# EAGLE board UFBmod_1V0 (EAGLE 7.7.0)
DL0WH Antenna BiTuner
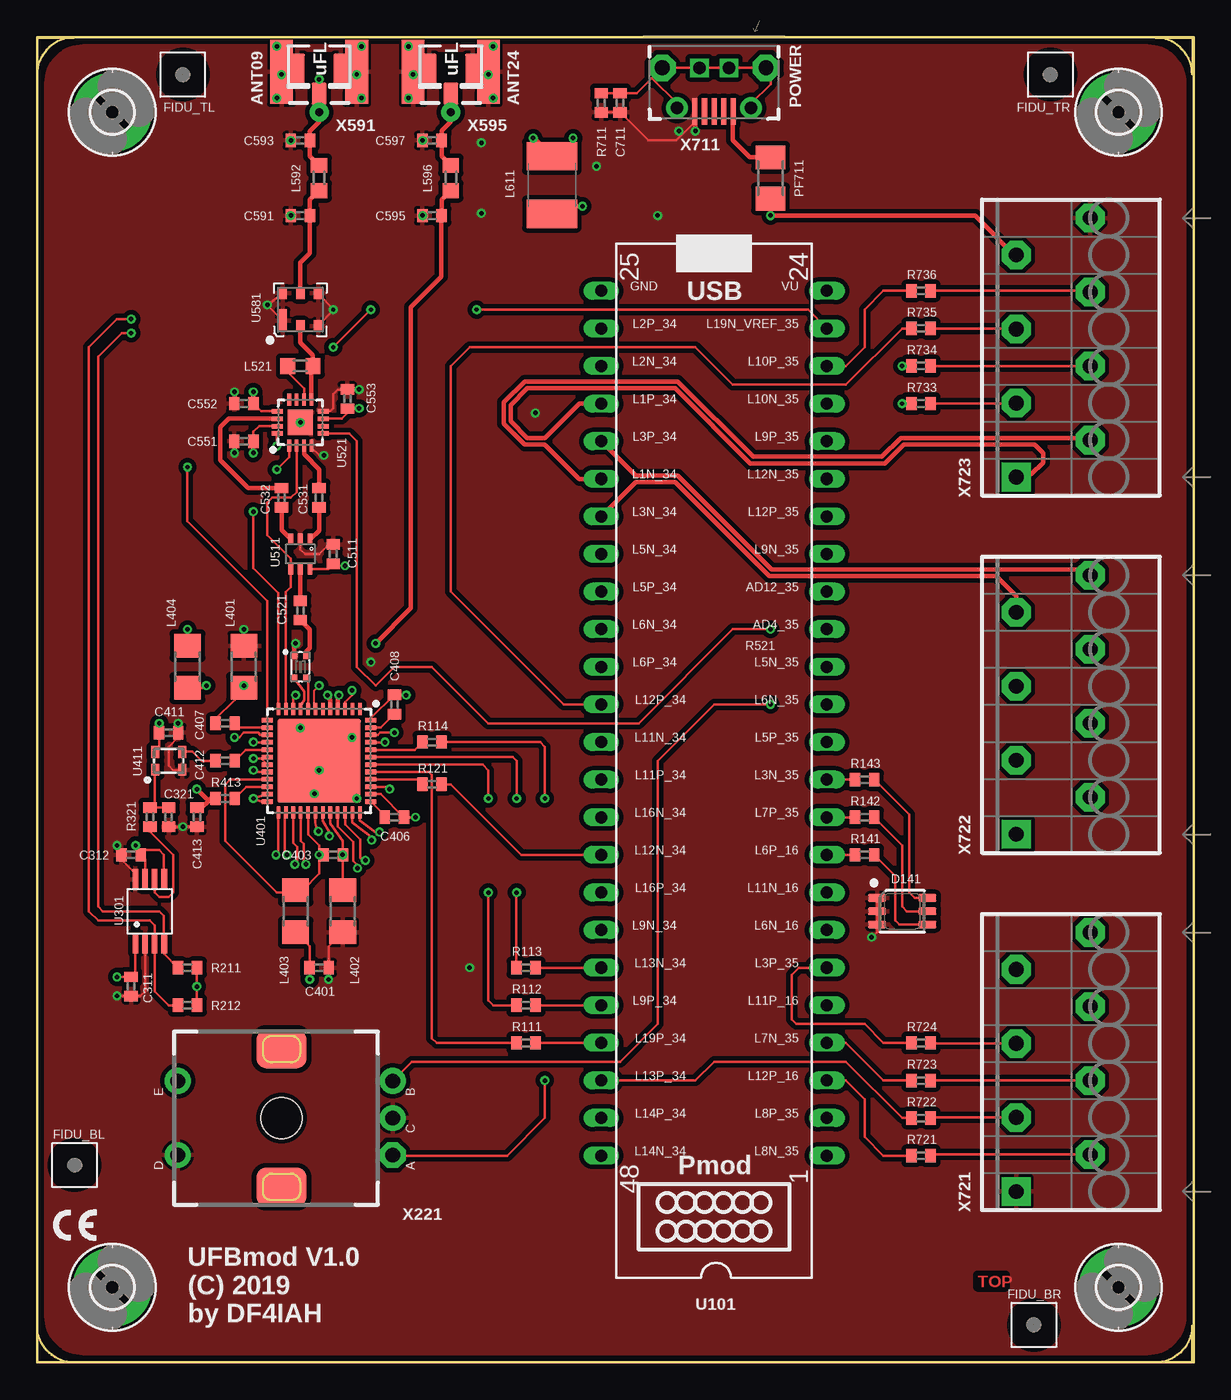
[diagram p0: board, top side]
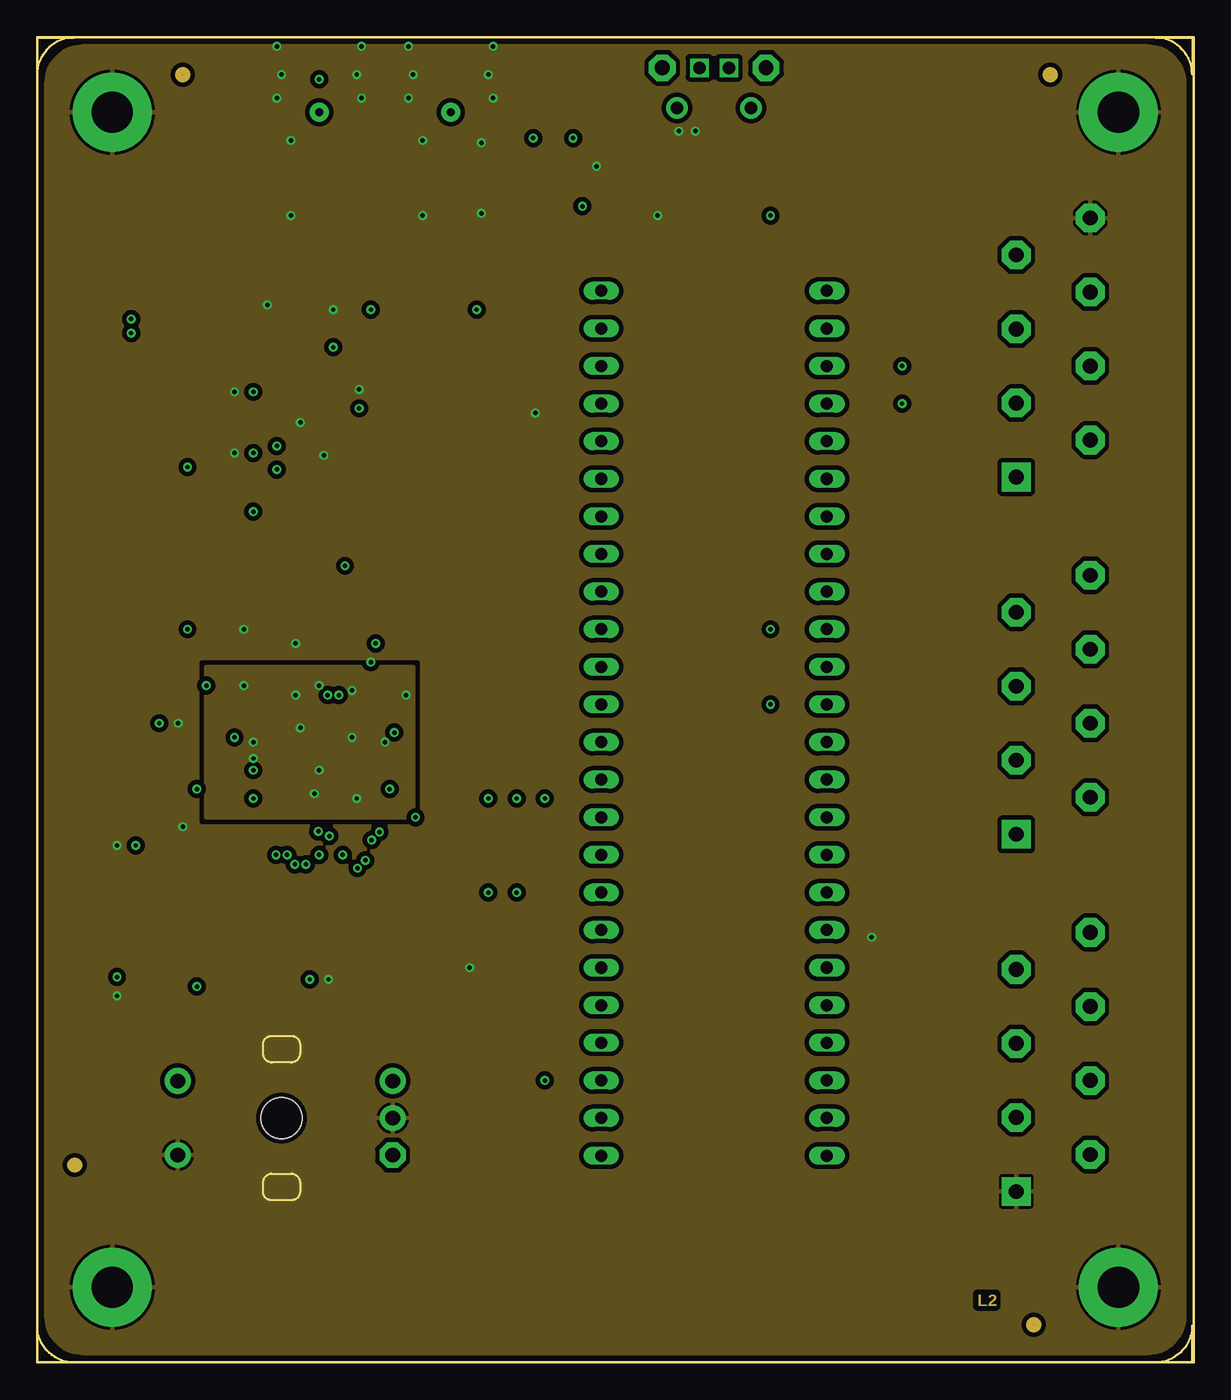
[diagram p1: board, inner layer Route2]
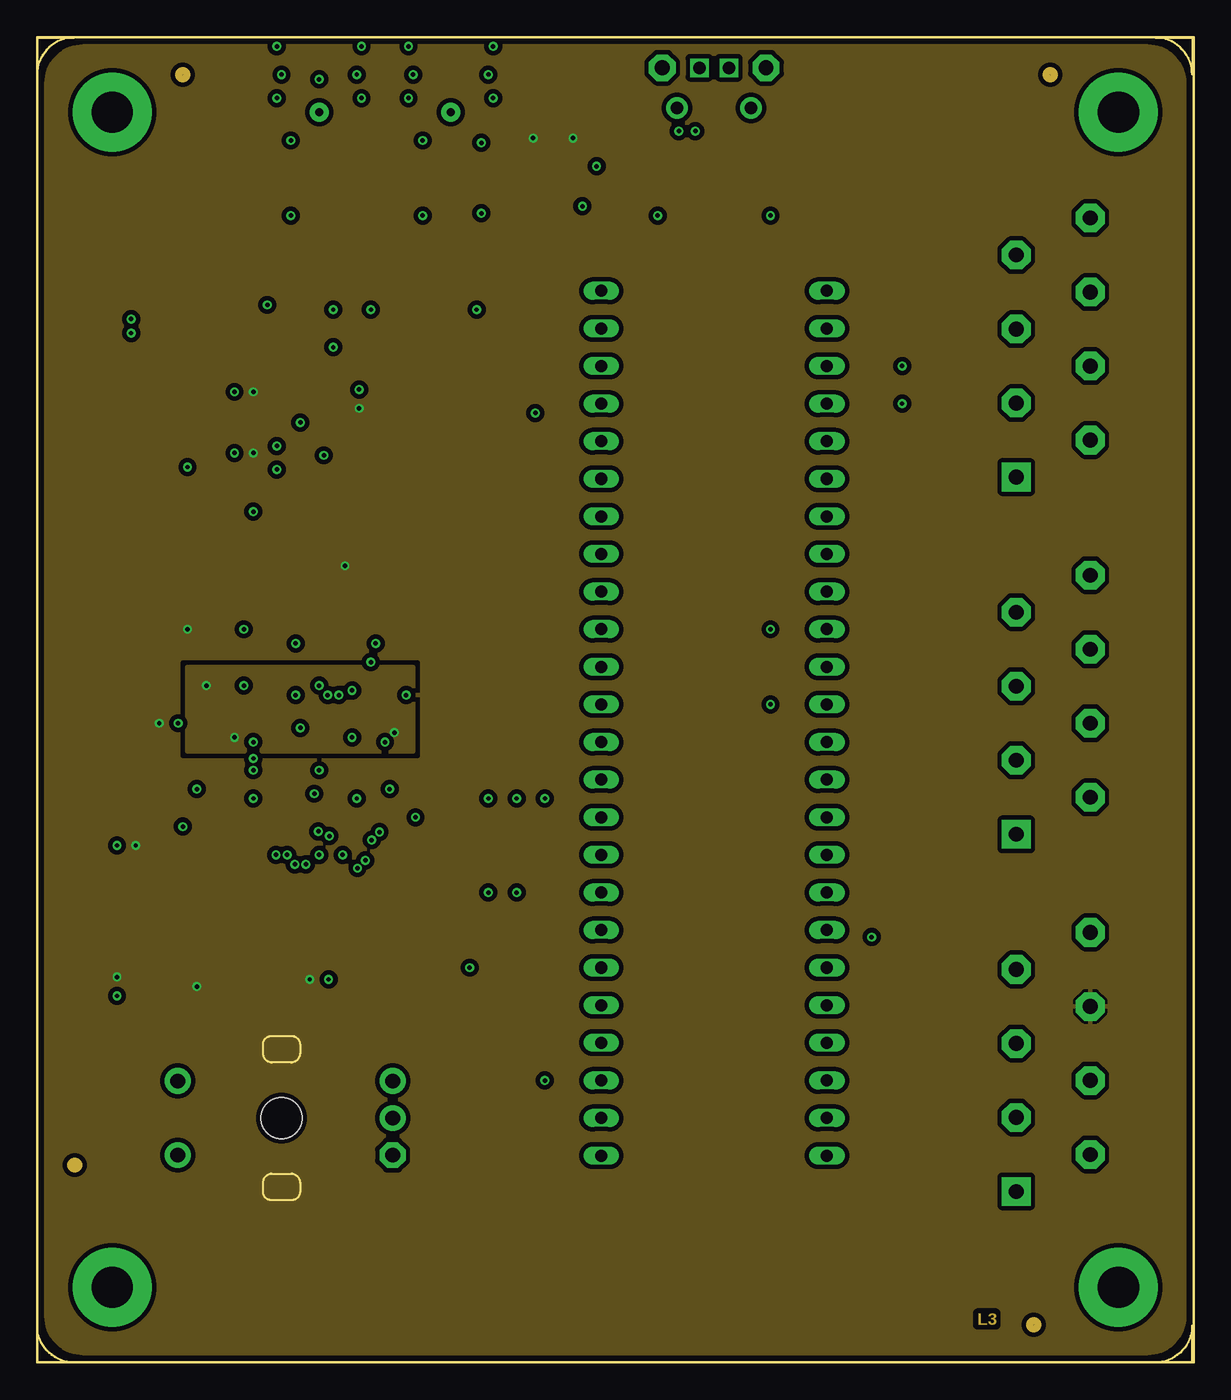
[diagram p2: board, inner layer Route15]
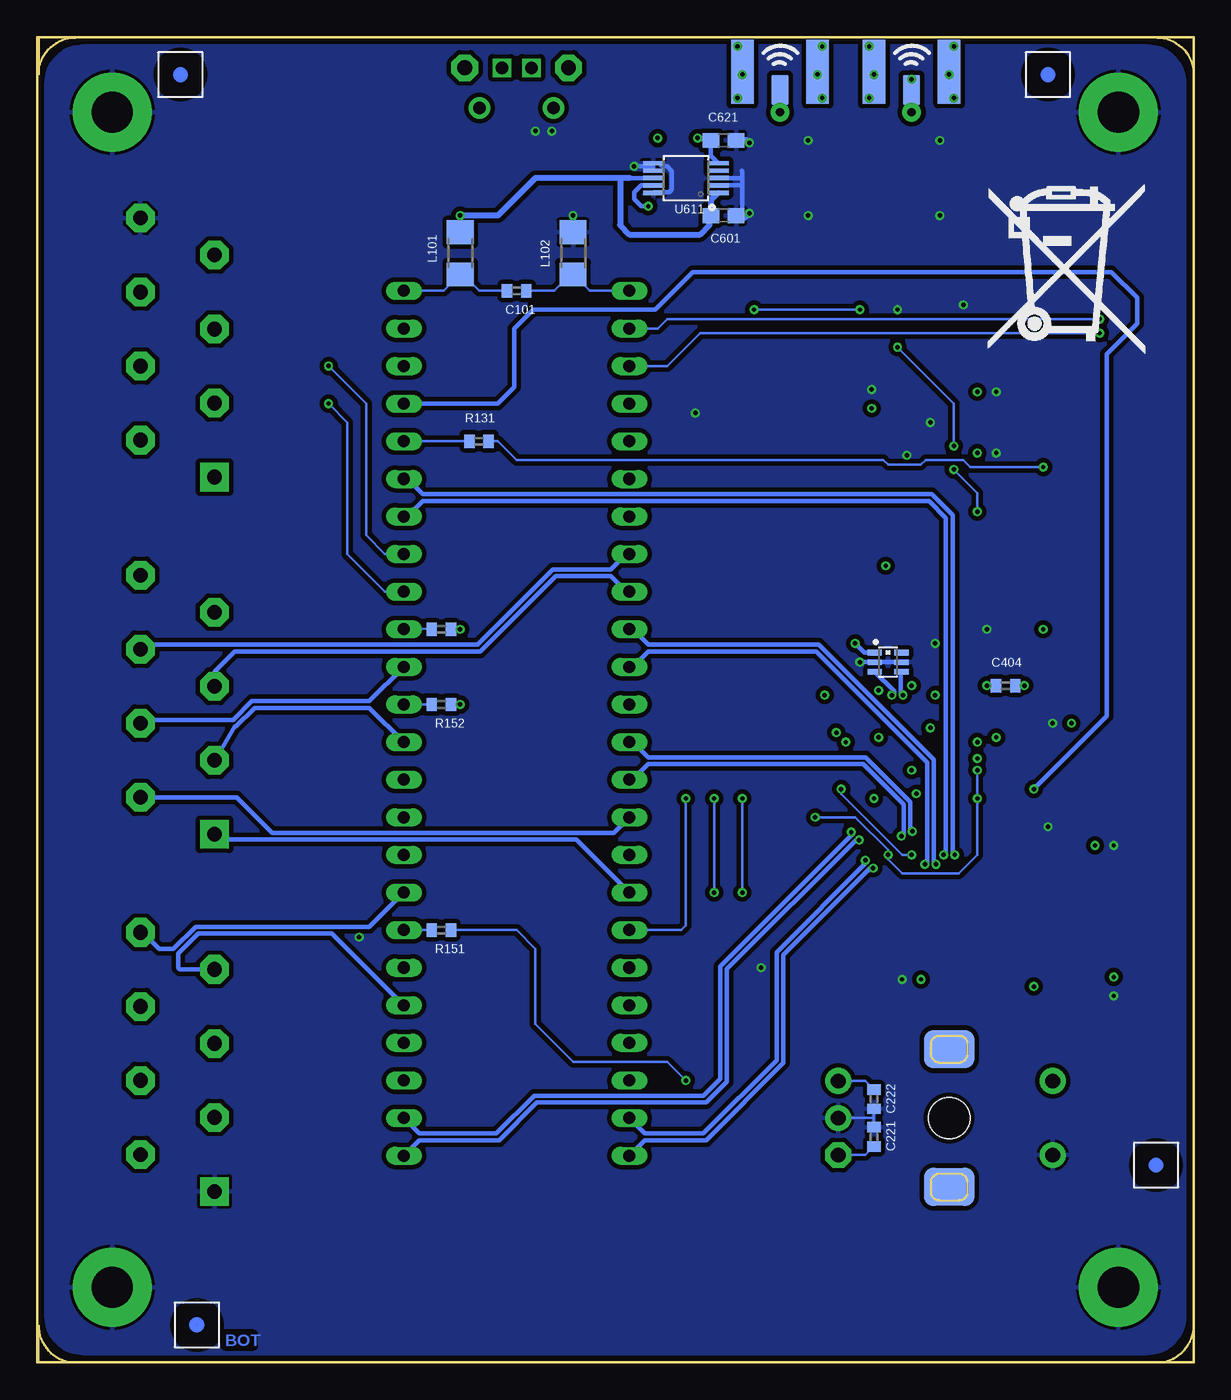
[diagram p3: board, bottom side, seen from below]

Size 78.11 x 89.53 mm. Coordinates in mm from the lower left corner, seen from the top.
Outline: 0,0 0,89.53 78.11,89.53 78.11,0 0,0
Copper layers (1+2*15+16): Top 0.035mm / dielectric 0.38mm / Route2 0.035mm / dielectric 0.71mm / Route15 0.035mm / dielectric 0.38mm / Bottom 0.035mm
Design rules "PCB-POOL Standard_ML4": minimum track width 0.15mm, minimum drill 0.3mm, track to track 0.15mm, track to pad 0.15mm, pad to pad 0.15mm, via to via 0.15mm, smd to smd 0.15mm, copper to edge 0.3mm, drill to drill 0.2mm, minimum pad ring 0.2mm, minimum via ring 0.15mm, stop-mask expansion 0.075mm, vias tented up to drill 0mil, thermal gap 0.2mm
Net classes: 0 default: drill 0.3 mm; 1 diff_100R: width 0.3 mm, clearance 0.15 mm; 2 pwr_ttl: width 0.75 mm, clearance 0.5 mm; 3 usb_pair: width 0.254 mm, clearance 0.152 mm; 4 pwrA5: width 0.4 mm; 5 single50R: width 0.838 mm, clearance 0.152 mm; 6 mil6_nofill: width 0.152 mm, clearance 0.254 mm
tRestrict: area 88.3,43.2 to 91.7,43.4; area 88.3,41.7 to 91.8,41.9; area 84.3,15.9 to 91.9,32.3
bRestrict: area 84.5,15.9 to 91.4,32.4; area 88.3,43.2 to 91.8,43.5; area 88.3,41.6 to 91.7,41.9; area 84.3,15.9 to 91.9,32.3
Milling: area 0,87 to 2.5,89.5; area 0,0 to 2.5,2.5; area 75.5,0 to 78,2.5; area 75.5,87 to 78,89.5

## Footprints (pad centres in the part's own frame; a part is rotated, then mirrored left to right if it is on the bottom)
C0402 = smd 0.7 x 0.9: 1 -0.65,0; 2 0.65,0
C0603 = smd 1.1 x 1: 1 -0.85,0; 2 0.85,0
ASMT-YTB7_0AA02_RGB = smd 1.2 x 0.5: 1 -1.7,0.9; 2 -1.7,0; 3 -1.7,-0.9; 4 1.7,-0.9; 5 1.7,0; 6 1.7,0.9
2,8-PAD = drill 2.8 pad 5.334: B2,8 0,0
R1206 = smd 1.6 x 1.803: 1 -1.422,0; 2 1.422,0
DXW21HN5011BL = smd 0.5 x 0.45: 1 -0.775,-0.4; 2 0.775,-0.4; 3 0.775,0.4; 4 -0.775,0.4
2450BL15B050 = smd 0.35 x 1: 1 -0.65,-0.9; 2 0,-0.9; 3 0.65,-0.9; 4 0.65,0.9; 5 0,0.9; 6 -0.65,0.9
L0603 = smd 1 x 1.1: 1 -0.85,0; 2 0.85,0
L1812 = smd 1.9 x 3.4: 1 -1.95,0; 2 1.95,0
M1206 = smd 1.6 x 2: 1 -1.4,0; 2 1.4,0
R0402 = smd 0.7 x 0.9: 1 -0.65,0; 2 0.65,0
DIGILENT_CMOD_A7__DIP48 = drill 0.813 long: 1 -29.21,-7.62; 2 -26.67,-7.62; 3 -24.13,-7.62; 4 -21.59,-7.62; 5 -19.05,-7.62; 6 -16.51,-7.62; 7 -13.97,-7.62; 8 -11.43,-7.62; 9 -8.89,-7.62; 10 -6.35,-7.62; 11 -3.81,-7.62; 12 -1.27,-7.62; 13 1.27,-7.62; 14 3.81,-7.62; 15 6.35,-7.62; 16 8.89,-7.62; 17 11.43,-7.62; 18 13.97,-7.62; 19 16.51,-7.62; 20 19.05,-7.62; 21 21.59,-7.62; 22 24.13,-7.62; 23 26.67,-7.62; 24 29.21,-7.62; 25 29.21,7.62; 26 26.67,7.62; 27 24.13,7.62; 28 21.59,7.62; 29 19.05,7.62; 30 16.51,7.62; 31 13.97,7.62; 32 11.43,7.62; 33 8.89,7.62; 34 6.35,7.62; 35 3.81,7.62; 36 1.27,7.62; 37 -1.27,7.62; 38 -3.81,7.62; 39 -6.35,7.62; 40 -8.89,7.62; 41 -11.43,7.62; 42 -13.97,7.62; 43 -16.51,7.62; 44 -19.05,7.62; 45 -21.59,7.62; 46 -24.13,7.62; 47 -26.67,7.62; 48 -29.21,7.62
µMAX8 = smd 1.35 x 0.4: 1 -2.15,0.975; 2 -2.15,0.325; 3 -2.15,-0.325; 4 -2.15,-0.975; 5 2.15,-0.975; 6 2.15,-0.325; 7 2.15,0.325; 8 2.15,0.975
QFN48_7X7-0P5-PAD = smd 0.8 x 0.3: 1 -3.5,2.75; 2 -3.5,2.25; 3 -3.5,1.75; 4 -3.5,1.25; 5 -3.5,0.75; 6 -3.5,0.25; 7 -3.5,-0.25; 8 -3.5,-0.75; 9 -3.5,-1.25; 10 -3.5,-1.75; 11 -3.5,-2.25; 12 -3.5,-2.75; 25 3.5,-2.75; 26 3.5,-2.25; 27 3.5,-1.75; 28 3.5,-1.25; 29 3.5,-0.75; 30 3.5,-0.25; 31 3.5,0.25; 32 3.5,0.75; 33 3.5,1.25; 34 3.5,1.75; 35 3.5,2.25; 36 3.5,2.75 | smd 0.3 x 0.8: 13 -2.75,-3.5; 14 -2.25,-3.5; 15 -1.75,-3.5; 16 -1.25,-3.5; 17 -0.75,-3.5; 18 -0.25,-3.5; 19 0.25,-3.5; 20 0.75,-3.5; 21 1.25,-3.5; 22 1.75,-3.5; 23 2.25,-3.5; 24 2.75,-3.5; 37 2.75,3.5; 38 2.25,3.5; 39 1.75,3.5; 40 1.25,3.5; 41 0.75,3.5; 42 0.25,3.5; 43 -0.25,3.5; 44 -0.75,3.5; 45 -1.25,3.5; 46 -1.75,3.5; 47 -2.25,3.5; 48 -2.75,3.5 | smd 5.65 x 5.65: 49 0,0
ASVTX-13 = smd 0.6 x 0.8: 1 -0.9,-0.6; 2 0.9,-0.6; 3 0.9,0.6; 4 -0.9,0.6
SC-70_6-LEAD_2X1MM25_0P65 = smd 0.4 x 0.8: 1 -0.65,-1; 2 0,-1; 3 0.65,-1; 4 0.65,1; 5 0,1; 6 -0.65,1
QFN16-3X3-0P5-PAD = smd 0.8 x 0.3: 1 -1.55,0.75; 2 -1.55,0.25; 3 -1.55,-0.25; 4 -1.55,-0.75; 9 1.55,-0.75; 10 1.55,-0.25; 11 1.55,0.25; 12 1.55,0.75 | smd 0.3 x 0.8: 5 -0.75,-1.55; 6 -0.25,-1.55; 7 0.25,-1.55; 8 0.75,-1.55; 13 0.75,1.55; 14 0.25,1.55; 15 -0.25,1.55; 16 -0.75,1.55 | smd 1.7 x 1.7: 17 0,0
B3440_3MM-X-3MM = smd 0.65 x 1.55: 1 -1.2,-0.75 | smd 0.65 x 0.8: 2 0,-1.125; 3 1.2,-1.125; 4 1.2,1.125; 5 0,1.125; 6 -1.2,1.125
S-PDSO-G10 = smd 0.3 x 1.45: 1 -1,-2.2; 2 -0.5,-2.2; 3 0,-2.2; 4 0.5,-2.2; 5 1,-2.2; 6 1,2.2; 7 0.5,2.2; 8 0,2.2; 9 -0.5,2.2; 10 -1,2.2
TTE_EN11-HSM = drill 1 pad 1.75 octagon: A -2.5,-7.5 | drill 1 pad 1.75: B 2.5,-7.5; C 0,-7.5; D -2.5,7; E 2.5,7 | smd 2.6 x 3.4: GND11 -4.65,0; GND12 4.65,0 | smd 2.6 x 3.4 bottom: GND21 -4.65,0; GND22 4.65,0 | hole 2.8: 0,0
SMA_UFL_PAD_TINY = smd 1.524 x 1.016: ANT1 -3.843,0 | drill 0.559 pad 1.27: ANT2 -5.08,0 | smd 2.032 x 1.143 bottom: ANT3 -3.589,0 | smd 2.2 x 1.016: GND1 -2.223,1.47; GND2 -2.223,-1.47 | smd 4.318 x 1.524: GND3 -2.349,-2.54; GND4 -2.349,2.54 | smd 4.318 x 1.524 bottom: GND5 -2.349,2.54; GND6 -2.349,-2.54
USB-B-MICRO-SMD_MOLEX-105017-0001 = smd 0.35 x 1.8: D+ 0,4.4; D- -0.65,4.4; GND 1.3,4.4; ID 0.65,4.4; VBUS -1.3,4.4 | drill 0.85 pad 1.45: JSHIELD -2.5,4.15; JSHIELD@2 2.5,4.15 | drill 1 pad 1.8 octagon: JSHIELD@3 -3.5,1.45; JSHIELD@6 3.5,1.45 | drill 0.85 square: JSHIELD@4 -1,1.45; JSHIELD@5 1,1.45
PHOENIX_1990067_1X8X2MM50_PTSA-0-5 = drill 1 pad 1.93 square: 1 -7.5,5 | drill 1 pad 1.93 octagon: 2 -5,0; 3 -2.5,5; 4 0,0; 5 2.5,5; 6 5,0; 7 7.5,5; 8 10,0

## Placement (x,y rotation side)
C101  100nF  [C0402]  45.72,72.39 180 bottom
C221  1nF  [C0402]  21.59,15.24 90 bottom
C222  1nF  [C0402]  21.59,17.78 270 bottom
C311  100nF  [C0402]  6.35,25.4 270 top
C312  100nF  [C0402]  6.35,34.29 180 top
C321  1uF  [C0402]  8.89,36.83 270 top
C401  1uF  [C0402]  19.05,26.67 0 top
C403  1nF  [C0402]  20,34.29 0 top
C404  1nF  [C0402]  12.7,45.72 180 bottom
C406  100nF  [C0402]  24.13,36.83 180 top
C407  100nF  [C0402]  12.7,43.18 0 top
C408  100nF  [C0402]  24.13,44.45 270 top
C411  10nF  [C0402]  8.89,42.55 0 top
C412  10nF  [C0402]  12.7,40.64 0 top
C413  56pF  [C0402]  10.79,36.83 270 top
C511  100nF  [C0402]  20,54.61 90 top
C521  1nF  [C0402]  17.78,50.8 270 top
C531  1nF  [C0402]  19.05,58.42 270 top
C532  1nF  [C0402]  16.51,58.42 270 top
C551  100nF  [C0402]  13.97,62.23 180 top
C552  100nF  [C0402]  13.97,64.77 180 top
C553  100nF  [C0402]  20.95,65.09 90 top
C591  0pF  [C0402]  17.78,77.47 180 top
C593  0pF  [C0402]  17.78,82.55 180 top
C595  0pF  [C0402]  26.67,77.47 180 top
C597  0pF  [C0402]  26.67,82.55 180 top
C601  10uF  [C0603]  31.75,77.47 0 bottom
C621  22uF  [C0603]  31.75,82.55 0 bottom
C711  1nF  [C0402]  39.37,85.09 90 top
D141  ASMT-YTB7-0AA02_RGB  [ASMT-YTB7_0AA02_RGB]  58.42,30.48 0 top
FIDU_BL  [FIDUCIAL_MARK_1MM]  2.54,13.34 0 top
FIDU_BR  [FIDUCIAL_MARK_1MM]  67.31,2.54 0 top
FIDU_TL  [FIDUCIAL_MARK_1MM]  9.84,87 0 top
FIDU_TR  [FIDUCIAL_MARK_1MM]  68.42,87 0 top
H2311  MOUNT-PAD-ROUND2.8  [2,8-PAD]  5.08,5.08 0 top
H2321  MOUNT-PAD-ROUND2.8  [2,8-PAD]  73.03,5.08 0 top
H2331  MOUNT-PAD-ROUND2.8  [2,8-PAD]  5.08,84.45 0 top
H2341  MOUNT-PAD-ROUND2.8  [2,8-PAD]  73.03,84.45 0 top
L101  300R  [R1206]  49.53,74.93 270 bottom
L102  300R  [R1206]  41.91,74.93 270 bottom
L401  300R  [R1206]  13.97,46.99 270 top
L402  300R  [R1206]  20.64,30.48 90 top
L403  300R  [R1206]  17.46,30.48 90 top
L404  300R  [R1206]  10.16,46.99 270 top
L421  MURATA DXW21HN5011BL  [DXW21HN5011BL]  17.78,46.99 270 top
L422  Johanson 2450BL15B050E  [2450BL15B050]  20.64,47.31 270 bottom
L521  ? nH  [L0603]  17.78,67.31 0 top
L592  0nH  [L0603]  19.05,80.01 90 top
L596  0nH  [L0603]  27.94,80.01 90 top
L611  10uH  [L1812]  34.77,79.53 270 top
PF711  1.1A/2.2A  [M1206]  49.53,80.01 90 top
R111  47R  [R0402]  33.02,21.59 180 top
R112  47R  [R0402]  33.02,24.13 180 top
R113  47R  [R0402]  33.02,26.67 180 top
R114  47R  [R0402]  26.67,41.91 180 top
R121  47R  [R0402]  26.67,39.05 180 top
R131  47R  [R0402]  48.26,62.23 180 bottom
R141  180R  [R0402]  55.88,34.29 180 top
R142  130R  [R0402]  55.88,36.83 180 top
R143  130R  [R0402]  55.88,39.37 180 top
R151  1kR  [R0402]  50.8,29.21 180 bottom
R152  1kR  [R0402]  50.8,44.45 180 bottom
R211  3.9kR  [R0402]  10.16,26.67 0 top
R212  3.9kR  [R0402]  10.16,24.13 0 top
R321  100kR  [R0402]  7.62,36.83 90 top
R413  100R  [R0402]  12.7,38.1 0 top
R521  1kR  [R0402]  50.8,49.53 180 bottom
R711  330kR  [R0402]  38.1,85.09 90 top
R721  100R  [R0402]  59.69,13.97 0 top
R722  100R  [R0402]  59.69,16.51 0 top
R723  100R  [R0402]  59.69,19.05 0 top
R724  100R  [R0402]  59.69,21.59 0 top
R733  100R  [R0402]  59.69,64.77 0 top
R734  100R  [R0402]  59.69,67.31 0 top
R735  100R  [R0402]  59.69,69.85 0 top
R736  100R  [R0402]  59.69,72.39 0 top
U101  DIGILENT_CMOD_A7  [DIGILENT_CMOD_A7__DIP48]  45.72,43.18 90 top
U301  MAX5217  [µMAX8]  7.62,30.48 90 top
U401  AT86RF215-ZU  [QFN48_7X7-0P5-PAD]  19.05,40.64 270 top
U411  ASVTX-13-D-26.000MHZ-I05-T  [ASVTX-13]  8.89,40.64 0 top
U511  PE4259  [SC-70_6-LEAD_2X1MM25_0P65]  17.78,54.61 180 top
U521  RFX1010  [QFN16-3X3-0P5-PAD]  17.78,63.5 90 top
U581  B39871B3440U410  [B3440_3MM-X-3MM]  17.78,71.12 0 top
U611  TPS62056DGSR  [S-PDSO-G10]  34.29,80.01 90 bottom
X221  TTE_EN11-HSM  [TTE_EN11-HSM]  16.51,16.51 90 top
X591  ANTENNATINY  [SMA_UFL_PAD_TINY]  19.05,89.53 90 top
X595  ANTENNATINY  [SMA_UFL_PAD_TINY]  27.94,89.53 90 top
X711  MOLEX 105017-0001  [USB-B-MICRO-SMD_MOLEX-105017-0001]  45.72,88.9 180 top
X721  PHOENIX_1990067_1X8X2MM50_PTSA-0-5  [PHOENIX_1990067_1X8X2MM50_PTSA-0-5]  71.12,19.05 90 top
X722  PHOENIX_1990067_1X8X2MM50_PTSA-0-5  [PHOENIX_1990067_1X8X2MM50_PTSA-0-5]  71.12,43.18 90 top
X723  PHOENIX_1990067_1X8X2MM50_PTSA-0-5  [PHOENIX_1990067_1X8X2MM50_PTSA-0-5]  71.12,67.31 90 top

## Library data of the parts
C101 C221 C222 C311 C312 C321 C401 C403 C404 C406-C408 C411-C413 C511 C521 C531 C532 C551-C553 C591 C593 C595 C597 C601 C621 C711 L101 L102 L401-L404 L521 L592 L596 L611 R111-R114 R121 R131 R141-R143 R151 R152 R211 R212 R321 R413 R521 R711 R721-R724 R733-R736 = df4iah_rcl
D141 = df4iah_led
FIDU_BL FIDU_BR FIDU_TL FIDU_TR = df4iah_fiducial
H2311 H2321 H2331 H2341 = df4iah_holes
L421 L422 = df4iah_balun
PF711 = rcl
U101 = df4iah_fpga
U301 = df4iah_dac
U401 U511 U521 U581 = df4iah_rf
U411 = df4iah_osc
U611 = df4iah_powersupply
X221 = df4iah_switch
X591 X595 = _c2h
X711 X721-X723 = df4iah_connector

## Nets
26MHZ_DAC_OUT: R321.1 U301.6
+3V3: C311.1 C312.1 C401.1 C411.1 C511.1 C551.1 C552.1 C553.1 C621.1 L403.1 L404.1 L611.1 R211.2 R212.2 U301.1 U301.5 U301.7 U411.4 U511.6 U521.7 U521.13 U521.15 U611.5 X721.6
+5V: C601.1 L101.1 PF711.1 U611.1 U611.8 X723.7
ANT09: C593.1 L592.2 X591.ANT1 X591.ANT2 X591.ANT3
ANT09_MATCH: C591.1 L592.1 U581.5
ANT24: C597.1 L596.2 X595.ANT1 X595.ANT2 X595.ANT3
FE09_ANT: L521.2 U521.9 U581.2
FE09_DET: R521.1 U521.5
FE09_IND: L521.1 U521.10
FE09_MODE: U101.23 U521.16
FE09_RX: C532.1 U521.14
FE09_TX: C531.1 U521.3
FPGA_1_34_N: U101.30 X723.2
FPGA_1_34_P: U101.28 X723.1
FPGA_3_34_N [diff_100R]: U101.29 X722.8
FPGA_3_34_P [diff_100R]: U101.31 X722.7
FPGA_3P35 [diff_100R]: R724.1 U101.6
FPGA_3P35_R [diff_100R]: R724.2 X721.5
FPGA_5_34_N [diff_100R]: U101.32 X722.6
FPGA_5_34_P [diff_100R]: U101.33 X722.5
FPGA_5_35_N [diff_100R]: U101.14 X722.4
FPGA_5_35_P [diff_100R]: U101.12 X722.3
FPGA_7N35 [diff_100R]: R723.1 U101.4
FPGA_7N35_R [diff_100R]: R723.2 X721.4
FPGA_9N35: R734.1 U101.17
FPGA_9N35_R: R734.2 X723.4
FPGA_10P35: R736.1 U101.22
FPGA_10P35_R: R736.2 X723.6
FPGA_11_16_N [diff_100R]: U101.8 X721.8
FPGA_11_16_P [diff_100R]: U101.5 X721.7
FPGA_12P16 [diff_100R]: R721.1 U101.3
FPGA_12P16_R [diff_100R]: R721.2 X721.2
FPGA_12P34: R735.1 U101.36
FPGA_12P34_R: R735.2 X723.5
FPGA_13P_34 [diff_100R]: R722.1 U101.46
FPGA_13P_34_R [diff_100R]: R722.2 X721.3
FPGA_16_34_N [diff_100R]: U101.39 X722.2
FPGA_16_34_P [diff_100R]: U101.41 X722.1
FPGA_AD12: R733.1 U101.16
FPGA_AD12_R: R733.2 X723.3
FPGA_FE09_DET: R521.2 U101.15
FPGA_I2C_SCL: R212.1 U101.26 U301.3
FPGA_I2C_SDA: R211.1 U101.27 U301.4
FPGA_MISO: R114.1 U101.42
FPGA_MOSI: R113.1 U101.43
FPGA_SCLK: R111.1 U101.45
FPGA_SELN: R112.1 U101.44
FPGA_TRX_CLKO: C413.1 R413.1 U101.21
FPGA_TRX_IRQ: R121.1 U101.40
FPGA_TRX_RSTN: R131.2 U101.20
GND: C221.2 C222.2 C311.2 C312.2 C321.2 C401.2 C411.2 C413.2 C511.2 C551.2 C552.2 C553.2 C591.2 C593.2 C595.2 C597.2 C601.2 C621.2 C711.1 D141.1 D141.2 D141.3 H2311.B2,8 H2321.B2,8 H2331.B2,8 H2341.B2,8 L102.1 L401.1 L402.1 L421.1 L422.2 L422.5 R711.1 U301.2 U301.8 U411.2 U511.2 U521.4 U521.8 U521.17 U581.1 U581.3 U581.4 U581.6 U611.3 U611.6 U611.7 U611.10 X221.C X221.D X591.GND1 X591.GND2 X591.GND3 X591.GND4 X595.GND1 X595.GND2 X595.GND3 X595.GND4 X711.GND X721.1 X723.8
LED_B: D141.6 R143.1
LED_B_R: R143.2 U101.11
LED_G: D141.5 R142.1
LED_G_R: R142.2 U101.10
LED_R: D141.4 R141.1
LED_R_R: R141.2 U101.9
PE09_RF1: C531.2 U511.1
PE09_RF2: C532.2 U511.3
PE09_RFC: C521.1 U511.5
PMIC3V3_SW: L611.2 U611.9
ROT_I: R151.2 U101.7
ROT_I_R: C221.1 R151.1 X221.A
ROT_Q: R152.2 U101.13
ROT_Q_R: C222.1 R152.1 X221.B
TRX_AVDD0: C407.2 U401.14
TRX_AVDD1: C408.2 U401.47
TRX_AVSS: C404.2 C407.1 C408.1 L401.2 U401.3 U401.6 U401.7 U401.10 U401.16 U401.18 U401.19 U401.45 U401.48 U401.49
TRX_CLKO: R413.2 U401.22
TRX_DEVDD: C403.1 L403.2 U401.21 U401.29 U401.39
TRX_DVDD: C406.2 U401.37
TRX_DVSS: C403.2 C406.1 L402.2 U401.20 U401.23 U401.24 U401.32 U401.38
TRX_EVDD: C404.1 L404.2 U401.15 U401.46
TRX_FEA09: U401.11 U511.4 U521.2
TRX_FEA24: U401.1
TRX_FEB09: U401.12 U521.1
TRX_FEB24: U401.2
TRX_IRQ: R121.2 U401.40
TRX_MISO: R114.2 U401.44
TRX_MOSI: R113.2 U401.43
TRX_RF09: C521.2 L421.4
TRX_RF09_N [diff_100R]: L421.2 U401.9
TRX_RF09_P [diff_100R]: L421.3 U401.8
TRX_RF24: C595.1 L422.1 L596.1
TRX_RF24_N: L422.4 U401.5
TRX_RF24_P: L422.3 U401.4
TRX_RSTN: R131.1 U401.13
TRX_RXCLK_N [diff_100R]: U101.48 U401.33
TRX_RXCLK_P [diff_100R]: U101.47 U401.34
TRX_RXD09_N [diff_100R]: U101.37 U401.30
TRX_RXD09_P [diff_100R]: U101.38 U401.31
TRX_RXD24_N [diff_100R]: U101.1 U401.35
TRX_RXD24_P [diff_100R]: U101.2 U401.36
TRX_SCLK: R111.2 U401.41
TRX_SELN: R112.2 U401.42
TRX_TCXO: C412.2 U401.17
TRX_TXCLK_N [diff_100R]: U101.19 U401.25
TRX_TXCLK_P [diff_100R]: U101.18 U401.26
TRX_TXD_N [diff_100R]: U101.34 U401.27
TRX_TXD_P [diff_100R]: U101.35 U401.28
USB_SHIELD: C711.2 R711.2 X711.JSHIELD X711.JSHIELD@2 X711.JSHIELD@3 X711.JSHIELD@4 X711.JSHIELD@5 X711.JSHIELD@6
USB_VBUS: PF711.2 X711.VBUS
VCCA: C101.2 L101.2 U101.24
VCTCXO_OUT: C412.1 U411.3
VCTCXO_VC: C321.1 R321.2 U411.1
VSSA: C101.1 L102.2 U101.25

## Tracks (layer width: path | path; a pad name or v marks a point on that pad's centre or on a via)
26MHZ_DAC_OUT
  Top 0.152: U301.6 7.94,32.64 7.94,31.75 8.26,31.43 8.89,31.43 9.21,31.75 9.21,34.29 7.62,35.88 R321.1
+3V3  (via drill 0.3)
  Top 0.15: 34.61,81.76 arc45 34.69,81.56 L611.1 | C511.1 20.15,53.82 v20.8,53.82
  Top 0.152: L403.1 18.4,28.12 C401.1 18.4,26.05 v18.41,25.88 | R211.2 10.79,26.66 v10.79,25.4 10.79,24.14 R212.2 | v5.4,26.04 6.33,26.04 C311.1 6.64,26.34 U301.1 | U301.7 7.3,32.64 7.3,33.97 7,34.27 C312.1 7,34.62 | U301.5 8.57,32.65 8.57,34.29 8.26,34.61 7.3,34.61 7,34.62 | 7,34.62 6.7,34.92 v6.67,34.92 | v8.26,43.18 8.26,42.56 C411.1 8.24,41.49 U411.4 | L404.1 v10.16,49.53 | U511.6 19.65,53.61 C511.1 | U521.13 15.14,64.25 C552.1 | U521.15 14.99,63.25 14.61,62.87 14.61,62.24 C551.1 | U521.7 20.57,63.75 20.95,64.14 C553.1 20.97,64.45 v21.75,64.45
  Top 0.3: v14.61,65.56 14.61,64.78 C552.1 | v14.61,61.44 14.61,62.22 C551.1 | 34.61,81.76 35.08,82.23 36.04,82.23 36.2,82.39 v36.2,82.71
  Top 0.406: 34.61,81.76 34.45,81.76 v33.5,82.71
  Bottom 0.15: 32.54,82.55 C621.1
  Bottom 0.3: U611.5 32.6,81.52 C621.1
  Bottom 0.406: v33.5,82.71 32.7,82.71 32.54,82.55
  pour Route15 (isolate 0.305, rank 2): 74.97,0.64 3.13,0.64 arc-90 0.64,3.13 0.64,86.4 arc-90 3.13,88.9 74.97,88.9 arc-90 77.47,86.4 77.47,3.13 arc-90
+5V  (via drill 0.3)
  Top 0.3: PF711.1 v49.53,77.47 63.34,77.47 66,74.81 X723.7
  Bottom 0.15: 32.7,77.47 C601.1
  Bottom 0.3: L101.1 v49.53,77.47 | U611.8 38.1,80.01
  Bottom 0.406: 38.1,80.01 38.73,80.01 | 38.73,80.01 44.45,80.01 46.99,77.47 v49.53,77.47 | U611.1 32.6,78.5 C601.1 | 38.73,80.01 38.73,76.83 38.1,76.2 33.34,76.2 32.7,76.83 32.7,77.47
ANT09  (via drill 0.3)
  Top 0.3: C593.1 18.43,81.48 L592.2 | 18.41,82.56 18.41,83.19 19.05,83.82 X591.ANT2 X591.ANT1 v19.05,86.68
  Top 0.406: 18.41,82.56 C593.1
  Bottom 0.3: X591.ANT3 v19.05,86.68
ANT09_MATCH
  Top 0.3: C591.1 18.43,78.54 L592.1 | U581.5 17.78,74.3 18.41,74.93 18.41,77.45
  Top 0.406: 18.41,77.45 C591.1
ANT24
  Top 0.3: L596.2 27.32,81.48 C597.1 27.32,83.2 27.94,83.82 X595.ANT2 X595.ANT1
  Bottom 0.3: X595.ANT3 X595.ANT2
FE09_ANT
  Top 0.3: U521.9 18.53,67.21 | L521.2 18.63,68.05 17.78,68.9 U581.2
  Top 0.406: 18.53,67.21 L521.2
FE09_DET  (via drill 0.3)
  Top 0.152: v49.53,49.53 46.99,49.53 40.64,43.18 30.48,43.18 26.67,46.99 24.13,46.99 22.86,45.72 21.59,46.99 21.59,62.23 21.07,62.75 U521.5
  Bottom 0.152: R521.1 v49.53,49.53
FE09_IND
  Top 0.152: U521.10 18.03,65.79 16.93,66.89 L521.1
FE09_MODE  (via drill 0.3)
  Top 0.152: U101.23 52.07,71.12 v29.69,71.12 | v22.54,71.12 v20,68.58 | U521.16 16.19,62.71 v16.19,61.91
  Bottom 0.152: v29.69,71.12 v22.54,71.12 | v16.19,61.91 16.19,64.77 v20,68.58
FE09_RX
  Top 0.3: C532.1 14.27,59.07 12.38,60.96 12.38,63.18 12.95,63.75 U521.14
FE09_TX
  Top 0.3: U521.3 18.03,61.34 19.05,60.33 C531.1
FPGA_1_34_N
  Top 0.3: U101.30 36.6,59.69 34.29,62.01 32.93,62.01 31.52,63.41 31.52,64.86 32.93,66.27 43.27,66.27 48.35,61.19 57.06,61.19 58.33,62.45 70.97,62.45 X723.2
FPGA_1_34_P
  Top 0.3: U101.28 36.6,64.77 34.29,62.45 33.11,62.45 31.98,63.59 31.98,64.68 33.11,65.81 43.09,65.81 48.17,60.73 57.24,60.73 58.51,62.01 67.38,62.01 67.94,61.44 67.94,60.8 67.15,60.01 66.32,60.01 X723.1
FPGA_3_34_N
  Top 0.3: U101.29 40.41,59.91 43.27,59.91 49.62,53.56 70.73,53.56 X722.8
FPGA_3_34_P
  Top 0.3: U101.31 40.41,59.47 43.09,59.47 49.44,53.12 64.77,53.12 66.12,51.77 X722.7
FPGA_3P35
  Top 0.152: U101.6 51.44,26.67 50.96,26.19 50.96,23.18 51.28,22.86 55.88,22.86 57.15,21.59 R724.1
FPGA_3P35_R
  Top 0.152: 60.38,21.55 X721.5
  Top 0.3: R724.2 60.38,21.55
FPGA_5_34_N
  Bottom 0.3: U101.32 38.33,54.61 39.37,53.56 43.27,53.56 48.35,48.48 70.81,48.48 X722.6
FPGA_5_34_P
  Bottom 0.3: U101.33 38.33,52.07 39.37,53.12 43.09,53.12 48.17,48.03 64.77,48.03 66.12,46.69 X722.5
FPGA_5_35_N
  Bottom 0.3: U101.14 55.66,44.67 63.59,44.67 64.86,43.41 70.89,43.41 arc-90 X722.4
FPGA_5_35_P
  Bottom 0.3: U101.12 55.66,44.23 63.41,44.23 64.68,42.95 64.77,42.95 66.04,40.76 arc90 X722.3
FPGA_7N35
  Top 0.152: U101.4 54.61,21.59 57.15,19.05 R723.1
FPGA_7N35_R
  Top 0.152: R723.2 X721.4
FPGA_9N35  (via drill 0.3)
  Top 0.152: v58.42,67.31 R734.1
  Bottom 0.152: U101.17 54.61,54.61 55.88,55.88 55.88,64.77 v58.42,67.31
FPGA_9N35_R
  Top 0.152: R734.2 X723.4
FPGA_10P35
  Top 0.152: U101.22 54.61,67.31 55.88,68.58 55.88,71.12 57.15,72.39 R736.1
FPGA_10P35_R
  Top 0.152: R736.2 71.04,72.39
  Top 0.3: 71.04,72.39 X723.6
FPGA_11_16_N
  Bottom 0.3: U101.8 55.66,29.43 67.4,29.43 68.9,27.94 69.85,27.94 70.96,29.05 X721.8
FPGA_11_16_P
  Bottom 0.3: U101.5 58.2,28.98 67.22,28.98 68.58,27.62 68.58,26.67 68.46,26.55 X721.7
FPGA_12P16
  Top 0.152: U101.3 54.61,19.05 55.88,17.78 55.88,15.24 57.15,13.97 R721.1
FPGA_12P16_R
  Top 0.152: 60.42,14.05 X721.2
  Top 0.3: R721.2 60.42,14.05
FPGA_12P34
  Top 0.152: U101.36 35.56,44.45 27.94,52.07 27.94,67.31 29.21,68.58 44.45,68.58 46.99,66.04 54.61,66.04 58.42,69.85 R735.1
FPGA_12P34_R
  Top 0.152: R735.2 66.08,69.85
  Top 0.3: 66.08,69.85 X723.5
FPGA_13P_34
  Top 0.152: U101.46 44.45,19.05 45.72,20.32 54.61,20.32 58.42,16.51 R722.1
FPGA_13P_34_R
  Top 0.152: 60.38,16.55 X721.3
  Top 0.3: R722.2 60.38,16.55
FPGA_16_34_N
  Bottom 0.3: U101.39 39.15,35.78 62.23,35.78 64.62,38.18 X722.2
FPGA_16_34_P
  Bottom 0.3: U101.41 41.69,35.34 65.78,35.34 X722.1
FPGA_AD12  (via drill 0.3)
  Top 0.152: v58.42,64.77 R733.1
  Bottom 0.152: U101.16 54.61,52.07 57.15,54.61 57.15,63.5 v58.42,64.77
FPGA_AD12_R
  Top 0.152: R733.2 66.08,64.77 X723.3
FPGA_FE09_DET
  Bottom 0.15: R521.2 U101.15
FPGA_I2C_SCL  (via drill 0.3)
  Top 0.152: R212.1 8.89,24.13 7.95,25.07 U301.3 7.94,28.34 7.94,29.53 7.62,29.84 4.13,29.84 3.49,30.48 3.49,68.58 5.4,70.48 v6.35,70.48
  Bottom 0.152: U101.26 36.2,69.85 35.56,70.48 v6.35,70.48
FPGA_I2C_SDA  (via drill 0.3)
  Top 0.152: R211.1 8.6,27.59 U301.4 8.57,28.35 8.57,30.16 8.26,30.48 4.45,30.48 4.13,30.8 4.13,67.94 5.71,69.53 v6.35,69.53
  Bottom 0.152: U101.27 35.56,67.31 33.34,69.53 v6.35,69.53
FPGA_MISO  (via drill 0.3)
  Top 0.152: R114.1 33.97,41.91 34.29,41.59 v34.29,38.1
  Bottom 0.152: U101.42 34.61,29.21 34.29,29.53 v34.29,38.1
FPGA_MOSI
  Top 0.152: U101.43 R113.1
FPGA_SCLK
  Top 0.152: U101.45 R111.1
FPGA_SELN
  Top 0.152: U101.44 R112.1
FPGA_TRX_CLKO  (via drill 0.3)
  Top 0.152: R413.1 11.75,38.1 | 11.13,37.48 C413.1
  Top 0.3: 11.75,38.1 11.59,37.94 | 11.59,37.94 11.13,37.48 | v10.79,38.73 11.59,37.94
  Bottom 0.3: v10.79,38.73 5.87,43.66 5.87,68.1 3.81,70.17 3.81,71.91 5.56,73.66 33.81,73.66 36.35,71.12 44.61,71.12 45.88,69.85 45.88,65.88 46.99,64.77 U101.21
FPGA_TRX_IRQ
  Top 0.152: R121.1 27.94,39.05 32.7,34.29 U101.40
FPGA_TRX_RSTN
  Bottom 0.152: R131.2 U101.20
GND  (via drill 0.3)
  Top 0.152: X711.GND 44.42,83.79 43.18,82.55 41.26,82.55 C711.1 R711.1 | L402.1 19.7,28.12 C401.2 19.7,26.05 v19.68,25.88 | v5.4,24.77 6.33,24.77 C311.2 6.37,24.77 6.99,24.77 7.29,25.07 U301.2 | U301.8 6.64,33.04 5.7,33.99 C312.2 5.4,34.59 v5.4,34.92 | C321.2 C413.2 10.78,36.2 v9.84,36.2 | v9.53,43.18 9.53,42.56 C411.2 9.54,42.24 8.89,41.59 8.89,40.32 9.21,40.01 9.76,40.01 U411.2 | L401.1 v13.97,49.53 | U511.2 17.78,54.93 18.1,54.61 19.05,54.61 19.7,55.26 | U581.4 19.05,72.17 v20,71.12 19.05,70.06 U581.3 | U581.6 16.51,72.17 v15.56,71.44 15.63,71.37 U581.1 | U521.8 19.8,64.25 20,64.45 20,65.41 20.32,65.72 20.94,65.72 C553.2 21.57,65.74 v21.75,65.72 | U521.4 18.53,61.8 19.05,61.28 v19.37,61.28 | v17.14,77.47 C591.2 | v17.14,82.55 C593.2 | D141.1 D141.2 D141.3 56.72,29.1 v56.36,28.73
  Top 0.3: L421.1 17.38,48.49 v17.46,48.58 | 19.7,55.26 C511.2 | v13.34,65.56 13.34,64.78 C552.2 | v13.34,61.44 13.34,62.22 C551.2 | v16.19,88.9 16.19,87.5 X591.GND4 17.45,87.19 X591.GND1 | v16.51,87 16.19,86.68 v16.19,85.41 | v21.91,88.9 21.91,87.5 X591.GND3 20.65,87.19 X591.GND2 | v21.91,85.41 21.59,85.72 v21.59,87 | 44.42,83.79 44.45,83.76 v44.45,83.19 | X595.GND4 25.4,88.58 v25.08,88.9 | v25.08,85.41 25.4,85.72 v25.4,87 X595.GND4 | v30.8,85.41 30.8,86.68 v30.48,87 X595.GND3 | v30.8,88.9 30.8,87.5 X595.GND3 | X595.GND1 25.53,87.31 X595.GND4 | X595.GND2 30.35,87.31 X595.GND3
  Bottom 0.15: 31.43,80.01 U611.3
  Bottom 0.152: 41.91,76.52 v41.91,77.47 | C221.2 21.59,16.51 | 21.59,16.51 C222.2 | X221.C 21.59,16.51
  Bottom 0.3: v22.54,47.31 L422.2 L422.5 | C601.2 30.48,77.89 30.48,79.53 | 30.48,79.53 30.48,80.01 | 30.48,80.01 30.48,80.49 30.5,80.51 | 30.48,80.01 31.43,80.01 | 30.48,79.53 31.43,79.53 | U611.6 36.7,80.8 v37.78,80.8 | U611.10 36.44,79.06 35.4,79.06 35.24,79.22 35.24,80.49 35.56,80.8 35.88,80.8 36.08,81.01 U611.6 | U611.7 U611.6
  Bottom 0.406: v30,82.39 30.16,82.55 30.96,82.55 | v30,77.63 30.32,77.31 30.8,77.31
  other vias: 17.78,63.5 26.04,82.55 26.04,77.47 29.21,26.67 33.66,64.14 43.34,83.19
  pour Top (isolate 0.305): 74.97,0.64 3.13,0.64 arc-90 0.64,3.13 0.64,86.4 arc-90 3.13,88.9 74.97,88.9 arc-90 77.47,86.4 77.47,3.13 arc-90
  pour Route2 (isolate 0.305, rank 2): 74.97,0.64 3.13,0.64 arc-90 0.64,3.13 0.64,86.4 arc-90 3.13,88.9 74.97,88.9 arc-90 77.47,86.4 77.47,3.13 arc-90
  pour Bottom (isolate 0.305): 74.97,0.64 3.13,0.64 arc-90 0.64,3.13 0.64,86.4 arc-90 3.13,88.9 74.97,88.9 arc-90 77.47,86.4 77.47,3.13 arc-90
LED_B
  Top 0.152: D141.6 59.27,31.38 58.9,31.75 58.9,37 R143.1
LED_B_R
  Top 0.152: U101.11 R143.2
LED_G
  Top 0.152: D141.5 58.74,30.48 58.42,30.8 58.42,34.94 R142.1
LED_G_R
  Top 0.152: U101.10 R142.2
LED_R
  Top 0.152: D141.4 58.21,29.58 57.94,29.84 57.94,32.88 R141.1
LED_R_R
  Top 0.152: U101.9 R141.2
PE09_RF1
  Top 0.3: U511.1 18.46,55.61 19.05,56.2 C531.2
PE09_RF2
  Top 0.3: C532.2 16.51,56.23 U511.3
PE09_RFC
  Top 0.3: U511.5 C521.1
PMIC3V3_SW  (via drill 0.3)
  Top 0.3: L611.2 35.29,78.11 v36.83,78.11
  Bottom 0.3: U611.9 36.51,79.53 37.31,79.53 37.78,79.06 37.78,78.58 37.31,78.11 v36.83,78.11
ROT_I
  Bottom 0.152: U101.7 R151.2
ROT_I_R  (via drill 0.3)
  Top 0.152: X221.A 24.05,13.97 31.75,13.97 34.29,16.51 v34.29,19.05
  Bottom 0.152: C221.1 22.17,14.01 X221.A | v34.29,19.05 35.56,20.32 41.91,20.32 44.45,22.86 44.45,27.94 45.72,29.21 R151.1
ROT_Q
  Bottom 0.152: U101.13 R152.2
ROT_Q_R  (via drill 0.3)
  Top 0.152: X221.B 25.32,20.32 39.37,20.32 41.91,22.86 41.91,40.64 45.72,44.45 v49.53,44.45
  Bottom 0.152: C222.1 22.17,19.01 X221.B | v49.53,44.45 R152.1
TRX_AVDD0
  Top 0.152: U401.14 13.64,42.89 C407.2
TRX_AVDD1
  Top 0.152: C408.2 23.22,42.89 U401.47
TRX_AVSS  (via drill 0.3)
  Top 0.15: U401.6 U401.7 18.73,44.21 18.73,45.4 v19.05,45.72
  Top 0.152: U401.48 22.55,43.52 C408.1 24.46,45.1 v24.92,45.09 | U401.3 20.8,44.61 21.27,45.09 v21.27,45.4 | v21.59,38.1 v18.73,38.42 19.05,38.42 v19.05,40.01 U401.49 19.05,41.59 v17.78,42.86 20.64,42.86 v21.27,42.23 | U401.10 17.3,44.92 v17.46,45.09 | v13.97,45.72 L401.2 13.34,44.93 13.34,44.77 12.05,43.48 C407.1 | U401.45 23.48,41.89 v23.5,41.91 | U401.16 14.62,41.89 v14.61,41.91 | U401.18 15.46,40.8 v14.61,40.8 15.14,40.8 U401.19
  Bottom 0.152: C404.2 13.35,45.7 v13.97,45.72
  pour Route2 (isolate 0.305): 11.43,46.99 25.4,46.99 25.4,36.83 11.43,36.83
TRX_CLKO
  Top 0.152: U401.22 14.14,38.89 R413.2
TRX_DEVDD  (via drill 0.3)
  Top 0.152: U401.29 18.3,35.67 19.05,34.92 v19.05,34.29 | v19.05,34.29 C403.1 | v19.05,34.29 19.05,33.02 17.93,31.9 L403.2 17.31,31.75 16.19,31.75 12.7,35.24 12.7,39.05 13.04,39.39 U401.21 | U401.39 23.66,38.89 v23.81,38.73
  Bottom 0.152: v23.81,38.73 23.81,38.42 19.68,34.29 v19.05,34.29
TRX_DVDD
  Top 0.152: U401.37 23.48,36.96 C406.2
TRX_DVSS  (via drill 0.3)
  Top 0.152: C403.2 v20.64,34.29 | U401.38 23.22,38.39 C406.1 v25.56,36.83 | v20.64,34.29 L402.2 | U401.32 19.8,36.4 20.64,35.24 v20.64,34.29 | U401.20 14.72,39.89 v14.61,40.01 | U401.23 v14.61,38.1 14.63,38.07 15.13,37.89 U401.24
  Bottom 0.152: v25.56,36.83 22.86,36.83 20.64,34.61 v20.64,34.29 20.64,33.97 19.68,33.02 15.88,33.02 14.61,34.29 v14.61,38.1 v14.61,40.01
TRX_EVDD  (via drill 0.3)
  Top 0.152: L404.2 11.28,45.57 v11.43,45.72 | U401.46 23.02,42.39 23.18,42.55 v24.13,42.55 | v13.34,42.23 13.65,42.23 13.97,42.55 14.92,42.55 15.08,42.39 U401.15
  Bottom 0.152: C404.1 v11.43,45.72
  pour Route15 (isolate 0.305): 10.16,46.99 25.4,46.99 25.4,41.27 10.16,41.27
TRX_FEA09
  Top 0.152: U401.11 16.8,52.04 17.13,52.37 U511.4 17.13,54.31 15.56,55.88 15.56,58.1 15.88,58.42 17.14,58.42 17.53,58.8 U521.2
TRX_FEB09  (via drill 0.3)
  Top 0.152: U401.12 16.3,51.96 14.61,53.66 v14.61,57.47 | U521.1 17.03,61.16 v16.19,60.33
  Bottom 0.152: v16.19,60.33 14.61,58.74 v14.61,57.47
TRX_IRQ
  Top 0.152: U401.40 22.57,39.37 25.72,39.37 R121.2
TRX_MISO
  Top 0.152: R114.2 25.5,41.39 U401.44
TRX_MOSI  (via drill 0.3)
  Top 0.152: U401.43 32.13,40.89 32.38,40.64 v32.38,38.1 | R113.2 32.37,31.73 v32.38,31.75
  Bottom 0.152: v32.38,38.1 v32.38,31.75
TRX_RF09
  Top 0.152: L421.4 18.18,48.02
  Top 0.3: 18.18,48.02 18.41,48.26 18.41,49.52 C521.2
TRX_RF09_N
  Top 0.152: L421.2 18.03,45.34 18.03,44.77 17.8,44.38 U401.9
TRX_RF09_P
  Top 0.152: L421.3 18.32,46.13 18.32,44.77 18.3,44.43
  Top 0.3: 18.3,44.43 U401.8
TRX_RF24  (via drill 0.3)
  Top 0.3: L596.1 27.32,78.54 C595.1 27.3,77.45 27.3,73.34 25.24,71.28 25.24,50.96 v22.86,48.58
  Bottom 0.3: L422.1 22.24,47.96 v22.86,48.58
TRX_RF24_N  (via drill 0.3)
  Top 0.3: v19.63,45.09 19.78,45.09 19.78,44.77 19.8,44.74 U401.5
  Bottom 0.3: L422.4 19.78,46.62 19.78,45.09 v19.63,45.09
TRX_RF24_P  (via drill 0.3)
  Top 0.3: v20.38,45.09 20.23,45.09 20.3,45.01 U401.4
  Bottom 0.3: L422.3 20.23,45.35 20.23,45.09 v20.38,45.09
TRX_RSTN  (via drill 0.3)
  Top 0.152: U401.13 15.55,51.44 10.16,56.83 v10.16,60.48
  Bottom 0.152: v10.16,60.48 15.08,60.48 15.56,60.96 18.1,60.96 18.41,60.64 20.64,60.64 20.95,60.96 45.72,60.96 46.99,62.23 R131.1
TRX_RXCLK_N  (via drill 0.3)
  Top 0.152: U401.33 20.3,36.21 21.36,35.15 21.36,33.88 21.75,33.5
  Top 0.3: 21.75,33.5 v21.64,33.39
  Bottom 0.3: v21.64,33.39 21.75,33.5 27.71,27.53 27.71,20.23 32.93,15.02 37.05,15.02 U101.48
TRX_RXCLK_P  (via drill 0.3)
  Top 0.152: U401.34 20.8,36.35 21.82,35.34 21.82,34.07 22.07,33.81
  Top 0.3: 22.07,33.81 v22.17,33.92
  Bottom 0.3: v22.17,33.92 22.07,33.81 28.16,27.72 28.16,20.41 33.11,15.46 37.05,15.46 U101.47
TRX_RXD09_N  (via drill 0.3)
  Top 0.152: U401.30 18.8,36.44 18.89,36.04 18.89,35.98
  Top 0.3: 19.14,35.88 v18.99,35.88 18.89,35.98
  Bottom 0.3: U101.37 37.88,41.91 36.83,40.87 22.13,40.87 19.14,37.88 19.14,35.88 v18.99,35.88
TRX_RXD09_P  (via drill 0.3)
  Top 0.152: U401.31 19.3,36.58 19.74,35.82 v19.74,35.56
  Top 0.3: 19.59,35.56 v19.74,35.56
  Bottom 0.3: U101.38 37.88,39.37 36.83,40.41 22.32,40.41 19.59,37.69 19.59,35.56 v19.74,35.56
TRX_RXD24_N  (via drill 0.3)
  Top 0.152: U401.35 21.3,36.48 22.7,35.4
  Top 0.3: 22.7,35.4 v22.59,35.3
  Bottom 0.3: v22.59,35.3 22.7,35.4 31.52,26.58 31.52,18.96 32.93,17.55 44.36,17.55 46.9,15.02 52.3,15.02 U101.1
TRX_RXD24_P  (via drill 0.3)
  Top 0.152: U401.36 21.8,36.62 23.02,35.72
  Top 0.3: 23.02,35.72 v23.12,35.83
  Bottom 0.3: v23.12,35.83 23.02,35.72 31.98,26.76 31.98,19.14 33.11,18 44.54,18 47.08,15.46 52.3,15.46 U101.2
TRX_SCLK
  Top 0.152: U401.41 26.47,39.89 26.67,39.69 26.67,21.91 26.99,21.59 R111.2
TRX_SELN  (via drill 0.3)
  Top 0.152: U401.42 30.09,40.39 30.48,40.01 v30.48,38.1 | v30.48,31.75 30.48,24.45 30.8,24.13 R112.2
  Bottom 0.152: v30.48,38.1 v30.48,31.75
TRX_TCXO
  Top 0.152: U401.17 14.1,41.39 C412.2
TRX_TXCLK_N  (via drill 0.3)
  Top 0.152: 16.29,34.29 16.29,37.12 U401.25
  Top 0.3: 16.29,34.29 v16.14,34.29
  Bottom 0.3: U101.19 53.12,59.69 52.07,58.65 17.69,58.65 16.29,57.24 16.29,34.29 v16.14,34.29
TRX_TXCLK_P  (via drill 0.3)
  Top 0.152: 16.73,34.29 16.73,37.08 U401.26
  Top 0.3: 16.73,34.29 v16.89,34.29
  Bottom 0.3: U101.18 53.12,57.15 52.07,58.2 17.87,58.2 16.73,57.06 16.73,34.29 v16.89,34.29
TRX_TXD_N  (via drill 0.3)
  Top 0.152: U401.27 17.3,35.09 17.55,34.83 17.55,33.66
  Top 0.3: 17.55,33.66 v17.41,33.66
  Bottom 0.3: U101.34 37.88,49.53 36.83,48.48 25.31,48.48 17.55,40.73 17.55,33.66 v17.41,33.66
TRX_TXD_P  (via drill 0.3)
  Top 0.152: U401.28 17.8,35.22 18,35.02 18,33.66
  Top 0.3: 18,33.66 v18.16,33.66
  Bottom 0.3: U101.35 37.88,46.99 36.83,48.03 25.49,48.03 18,40.55 18,33.66 v18.16,33.66
USB_SHIELD
  Top 0.152: R711.2 C711.2 40.51,85.74 41.52,86.75 | 41.52,86.75 X711.JSHIELD@6 X711.JSHIELD@5 X711.JSHIELD@4 X711.JSHIELD@3 49.53,87.14 49.53,86.36 48.22,85.05 X711.JSHIELD | X711.JSHIELD@2 43.22,85.05 41.52,86.75
USB_VBUS
  Top 0.152: X711.VBUS 46.99,84.47
  Top 0.3: 46.99,84.47 46.99,82.55 48.13,81.41 PF711.2
VCCA
  Bottom 0.152: U101.24 50.65,72.39 L101.2 49.38,73.51 48.26,72.39 C101.2
VCTCXO_OUT
  Top 0.152: U411.3 9.82,41.27 10.48,41.27 11.11,40.64 C412.1
VCTCXO_VC
  Top 0.152: C321.1 R321.2 7.63,37.48 7.94,37.78 7.94,39.99 U411.1
VSSA
  Bottom 0.152: U101.25 40.79,72.39 L102.2 42.06,73.51 43.18,72.39 C101.1

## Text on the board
Top: TOP
Route2: L2
Route15: L3
Bottom: BOT
tPlace: ANT09 | ANT24 | POWER | UFBmod V1.0 / (C) 2019 / by DF4IAH
tNames: X591 | X595
tDocu: WDG20..WDG24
